(* Logix 5000 AddOnInstructionDefinition export MAS_Yaskawa; software revision 17.00 *)

TYPE Yaskawa_EIP_Servo :   // Yaskawa SigmaLogic Axis Structure v2.4.0
STRUCT
   O : Yaskawa_OUT_to_Servo;
   I : Yaskawa_IN_from_Servo;
   AOI_SB : Yaskawa_AOI_Status_Bits;
END_STRUCT
END_TYPE

TYPE Yaskawa_OUT_to_Servo :   // Structure of data sent out to the Yaskawa SigmaLogic controller v2.4.0
STRUCT
   b00_ServoOn : BOOL;   // Servo On
   b01_Stop : BOOL;   // Stops All Current Motion in Progress
   b02_Home : BOOL;   // Start Homing Process
   b03_MoveStart1 : BOOL;   // Start Current Motion
   b06_SuperImpose : BOOL;
   b07_ServoAlarmReset : BOOL;   // Servo Alarm Reset
   b08_ControllerAlarmReset : BOOL;   // SigmaLogic Alarm Reset
   b09_MoveStart2 : BOOL;   // Start Second Motion (Blended Move)
   b10_MoveAbort : BOOL;   // Abort Current Move
   b11_MovePause : BOOL;   // Pause Current Move
   b12_SeqPause : BOOL;   // Indexing Sequence Pause
   b13_SeqResume : BOOL;   // Indexing Sequence Resume
   b14_SeqCancel : BOOL;   // Indexing Sequence Cancel
   b15_AbsEncoderReset : BOOL;   // Absolute Encoder Reset
   b16_SeqStart : BOOL;   // Start Indexing Sequence
   b17_SeqEditSpeed : BOOL;   // Enter Edit Speed
   b18_SeqEditDistance : BOOL;   // Enter Distance Edit
   b19_PLSEnable : BOOL;   // Enable PLS execution
   b20_PLSActivateOutput1 : BOOL;   // Activate PLS output1 switch logic
   b21_PLSActivateOutput2 : BOOL;   // Activate PLS output2 switch logic
   b22_PLSActivateOutput3 : BOOL;   // Activate PLS output3 switch logic
   b23_PLSActivateOutput4 : BOOL;   // Activate PLS output4 switch logic
   b24_SetClock : BOOL;   // Set the remote controller clock with data provided by the PLC
   RebootController : BOOL;
   UseExternalEncoder : BOOL;   // Use External Encoder when executing MAHSP_Yaskawa
   b32_HeatbeatAnswer : BOOL;   // Heartbeat Answer
   BrakeBypassRequest : BOOL;
   SetFwdTorqueLimit : BOOL;
   SetRevTorqueLimit : BOOL;
   TorqueLimit : DINT;
   TorqueRamp : DINT;
   HomeMethod : INT;
   HomeSpeed : DINT;
   HomeAccDec : DINT;   // Home Move Acceleration/Deceleration Rate
   HomeBackOffDistance : DINT;
   HomeCreepSpeed : DINT;
   HomeCreepDistanceLimit : DINT;
   HomeCreepTimeLimit : DINT;
   HomeOffsetDistance : DINT;
   HomeOffsetSpeed : DINT;
   HomePostion : DINT;
   HomeTorque : DINT;
   HomeInputNo : DINT;
   HomeApproachTimeLimit : DINT;
   HomeApproachDistLimit : DINT;
   HomeDirection : INT;
   HomeSwitchMode : INT;
   MoveType : INT;
   MoveDirection : INT;
   MoveAccel1 : DINT;
   MoveAccel2 : DINT;
   MoveDecel1 : DINT;
   MoveDecel2 : DINT;
   MoveSpeed1 : DINT;
   MoveSpeed2 : DINT;
   MoveDistance1 : DINT;
   MoveDistance2 : DINT;
   MovePosition1 : DINT;
   MovePosition2 : DINT;
   RegistrationDistance : DINT;
   GearNumerator : DINT;
   GearDenominator : DINT;
   SuperImposeDistance : DINT;
   Resolution : INT;
   RegistrationDirection : INT;
   TuningLevel : INT;
   SequenceStep : INT;   // Staring Sequence Step Number
   SequenceEditStep : INT;   // Sequence Step Number to Edit
   FlagCommandBits1 : DINT;   // Flag Commands. 1..64 are General Flags, Bits 0..31 correspond to Flag 1..32
   FlagCommandBits2 : DINT;   // Flag Commands cont. 1..64 are General Flags, Bits 0..31 correspond to Flag 33..64
   DigitalOutCommandBits : DINT;   // Digital Output commands. Bits 0-7 correspond to CN13 Digital Outputs 0-7, used as Flag 73-80. Bits 8-10 correspond to CN1 Digital Outputs 0-2 used as Flag 88-90"
   SequenceEditSpeed : DINT;
   SequenceEditDistance : DINT;
   FeedRateOverride : INT;
   HSI_Enable : BOOL;
   HSI_MoveMode : BOOL;   // 0=Relative; 1=Moves per Cycle
   HSI_CalcMethod : BOOL;   // 0=Accel/Decel; 1=Time
   HSI_MoveDirection : BOOL;   // 0 = Negative; 1 = Positive
   HSI_TriggerFlag : INT;
   HSI_MovingFlag : INT;
   HSI_DwellingFlag : INT;
   HSI_DoneFlag : INT;
   HSI_MoveType : INT;   // 0=Single; 1=Repeat; 2=Repeat "x" times
   HSI_RepeatNumber : INT;
   HSI_Distance : DINT;
   HSI_Speed : DINT;
   HSI_Accel : DINT;
   HSI_MoveTime : DINT;
   HSI_DwellTime : DINT;
   PLS_OutputFlag1 : INT;
   PLS_OutputFlag2 : INT;
   PLS_OutputFlag3 : INT;
   PLS_OutputFlag4 : INT;
   PLS_OnPosition1 : DINT;
   PLS_OffPosition1 : DINT;
   PLS_OnPosition2 : DINT;
   PLS_OffPosition2 : DINT;
   PLS_OnPosition3 : DINT;
   PLS_OffPosition3 : DINT;
   PLS_OnPosition4 : DINT;
   PLS_OffPosition4 : DINT;
   PLS_OnCompensation1 : INT;
   PLS_OffCompensation1 : INT;
   PLS_OnCompensation2 : INT;
   PLS_OffCompensation2 : INT;
   PLS_OnCompensation3 : INT;
   PLS_OffCompensation3 : INT;
   PLS_OnCompensation4 : INT;
   PLS_OffCompensation4 : INT;
   RTC_Year : INT;
   RTC_Month : INT;
   RTC_Day : INT;
   RTC_Hour : INT;
   RTC_Min : INT;
   RTC_Sec : INT;
   StopDecel : DINT;
   AnalogOutput : INT;   // CN13, AO_01 [mV]
END_STRUCT
END_TYPE

TYPE Yaskawa_AOI_Status_Bits :   // Internal bits used to interlock Yaskawa AOI execution. v2.4.0
STRUCT
   MAM : BOOL;   // Move AOI Active
   MAJ : BOOL;   // Jog AOI Active
   MAB : BOOL;   // Blending AOI Active
   MAG : BOOL;   // Gearing AOI Active
   MAHSP : BOOL;   // Home SetPoint AOI Active
   MAH : BOOL;   // Homing AOI Active
   MSQE : BOOL;   // Sequence Edit AOI Active
   MSQR : BOOL;   // Sequence Run AOI Active
   MHSI : BOOL;   // High Speed Index AOI Active
   MSO : BOOL;   // Servo On
   MSF : BOOL;   // Servo Off
   MAFR : BOOL;   // Fault Reset
   MAS : BOOL;   // Servo Abort
   MTRQ : BOOL;   // Torque Mode Active
   MPLS : BOOL;   // PLS Active
   MCLK : BOOL;   // SetClock Active
   MSTL : BOOL;   // Set Torque Limit Active
   AOI_Permissive : BOOL;   // Permissive to Execute an AOI
END_STRUCT
END_TYPE

TYPE Yaskawa_IN_from_Servo :   // Structure of data coming from the Yaskawa SigmaLogic controller. v2.4.0
STRUCT
   AlarmText : STRING;   // ServoPack Alarm Code plus Text Description
   b00_Heartbeat : BOOL;
   b01_Alarm : BOOL;   // ServoPack Alarm
   b02_Warning : BOOL;   // ServoPack Warning
   b03_Ready : BOOL;   // ServoPack Ready
   b04_Enabled : BOOL;   // ServoPack Enabled ("Servo On")
   b05_StopComplete : BOOL;
   b06_HomeComplete : BOOL;
   b07_HomeBusy : BOOL;
   b08_HomeActive : BOOL;
   b09_HomeAborted : BOOL;
   b10_HomeError : BOOL;
   b11_MoveAbsComplete : BOOL;
   b12_MoveAbsBusy : BOOL;
   b13_MoveAbsActive : BOOL;
   b14_MoveAbsAborted : BOOL;
   b15_MoveAbsError : BOOL;
   b16_MoveRelComplete : BOOL;
   b17_MoveRelBusy : BOOL;
   b18_MoveRelActive : BOOL;
   b19_MoveRelAborted : BOOL;
   b20_MoveRelError : BOOL;
   b21_JogAtSpeed : BOOL;
   b22_JogBusy : BOOL;
   b23_JogActive : BOOL;
   b24_JogAborted : BOOL;
   b25_JogError : BOOL;
   b26_GearInSync : BOOL;
   b27_GearBusy : BOOL;
   b28_GearActive : BOOL;
   b29_GearAborted : BOOL;
   b30_GearError : BOOL;
   b32_MoveSuperComplete : BOOL;
   b33_MoveSuperBusy : BOOL;
   b34_MoveSuperActive : BOOL;
   b35_MoveSuperAborted : BOOL;
   b36_MoveSuperError : BOOL;
   b37_PowerCycleRequired : BOOL;
   b38_MoveBlend1Complete : BOOL;
   b39_MoveBlend1Busy : BOOL;
   b40_MoveBlend1Active : BOOL;
   b41_MoveBlend1Abort : BOOL;
   b42_MoveBlend1Error : BOOL;
   b43_MoveBlend2Complete : BOOL;
   b44_MoveBlend2Busy : BOOL;
   b45_MoveBlend2Active : BOOL;
   b46_MoveBlend2Abort : BOOL;
   b47_MoveBlend2Error : BOOL;
   b48_RegComplete : BOOL;
   b49_RegBusy : BOOL;
   b50_RegActive : BOOL;
   b51_RegAborted : BOOL;
   b52_RegError : BOOL;
   b53_ResetAbsEncoderActive : BOOL;
   b54_ResetAbsEncoderBusy : BOOL;
   b55_ResetAbsEncoderDone : BOOL;
   b56_ResetAbsEncoderError : BOOL;
   b57_SeqRunning : BOOL;
   b58_RegSensorNotReached : BOOL;
   b59_SeqEditError : BOOL;
   b60_SeqEditDone : BOOL;
   b61_TorqueAtTorque : BOOL;
   b62_TorqueBusy : BOOL;
   b63_TorqueActive : BOOL;
   b64_TorqueAborted : BOOL;
   b65_TorqueError : BOOL;
   b66_ControllerAlarm : BOOL;
   b67_ApplicationError : BOOL;
   b68_AxisAtStandStill : BOOL;
   b69_TestModeActive : BOOL;
   b70_ServoParamsOK : BOOL;
   b71_SetFwdTorqueLimitDone : BOOL;
   b72_SetRevTorqueLimitDone : BOOL;
   Position : DINT;
   Speed : DINT;
   Torque : DINT;
   HomeErrorID : INT;
   MoveAbsErrorID : INT;
   MoveRelErrorID : INT;
   JogErrorID : INT;
   GearErrorID : INT;
   MoveSuperErrorID : INT;
   ServoAlarmID : INT;
   ServoWarningID : INT;
   ControllerAlarmID : DINT;
   AxisGenAlarmID : DINT;
   MoveBlend1ErrorID : INT;
   MoveBlend2ErrorID : INT;
   ResetAbsEncoderErrorID : INT;
   FunctionBlockErrorID : INT;
   TorqueErrorID : INT;
   RegErrorID : INT;
   SeqCurrentStep : INT;
   FlagStatusBit1 : DINT;   // Flag Status. 1..64 are General Flags, Bits 0..31 correspond to Flag 1..32
   FlagStatusBit2 : DINT;   // Flag Status cont. 1..64 are General Flags, Bits 0..31 correspond to Flag 33..64
   IOStatusBits : DINT;   // Digital IO Status. Bits 0-7, CN13 Inputs 0-7, Used as Flag 65-72. Bits 8-15, CN13 Outputs 0-7, Used as Flag 73-80. Bits 16-22, CN1 Inputs 0-6, Used as Flag 81-87. Bits 23-25, CN1 Outputs 0-4, Used as Flag 88-92.
   HSI_Moving : BOOL;
   HSI_Dwelling : BOOL;
   HSI_Done : BOOL;
   HSI_Busy : BOOL;
   HSI_Error : BOOL;
   HSI_ErrorCode : INT;
   PLS_Running : BOOL;
   PLS_SwitchStatus1 : BOOL;
   PLS_SwitchStatus2 : BOOL;
   PLS_SwitchStatus3 : BOOL;
   PLS_SwitchStatus4 : BOOL;
   PLS_Busy : BOOL;
   PLS_Error : BOOL;
   PLS_ErrorCode : INT;
   SetClock_Done : BOOL;
   SetClock_Busy : BOOL;
   SetClock_Error : BOOL;
   SetClock_ErrorID : INT;
   SoftwareVersion : DINT;
   FirmwareVersion : DINT;
   CommandedPos : DINT;
   CommandedPosNonCyc : DINT;
   CommandedSpeed : DINT;
   Clock_Year : INT;
   Clock_Month : INT;
   Clock_Day : INT;
   Clock_Hour : INT;
   Clock_Minute : INT;
   Clock_Second : INT;
   AnalogInput : REAL;   // CN13, AI_01 [v]
   BrakeBypassActive : BOOL;
   ForwardTorqueLimit : DINT;
   ReverseTorqueLimit : DINT;
END_STRUCT
END_TYPE

ADD_ON_INSTRUCTION MAS_Yaskawa   (* revision 2.4 0, vendor Yaskawa America, Inc., ExecuteEnableInFalse *)
// Motion Axis Stop
// Revision note:
// 2.4.0: No functional change
// 2.3.1: Moved unlatch of AOI_ON_LOCAL to bottom of EnableInFalse routine so that outputs will be on for at least 1 scan if one-shot on EN is used.
// 2.3.0: No functional change
// 2.0.0: Added IP output for stopping in progress. Improved output operation. Improved interlocking with embedded code.
// 1.2.0: No functional change.
// Initial Release 9/10/2014
// Help:
// This AOI stops any motion in progress on the servo axis on the rising edge of the EnableIN input. The Deceleration rate specified with this AOI will be used during stopping. If Deceleration is left at zero, the rate will default to 1000 units/s/s
VAR_IN_OUT
   Axis : Yaskawa_EIP_Servo; {required}
END_VAR
VAR_INPUT
   Deceleration : REAL; {required}   // The Deceleration rate used during stopping.
END_VAR
VAR_OUTPUT
   EN : BOOL; {visible}   // The AOI is Active
   IP : BOOL; {visible}   // The axis is in the process of stopping
   PC : BOOL; {visible}   // Motion is successfully stopped/aborted
END_VAR
VAR
   AOI_ON_LOCAL : BOOL;
   ScaleFactor : REAL;
   Finished : BOOL;   // The Function is finished
END_VAR

ROUTINE EnableInFalse   (* ladder *)
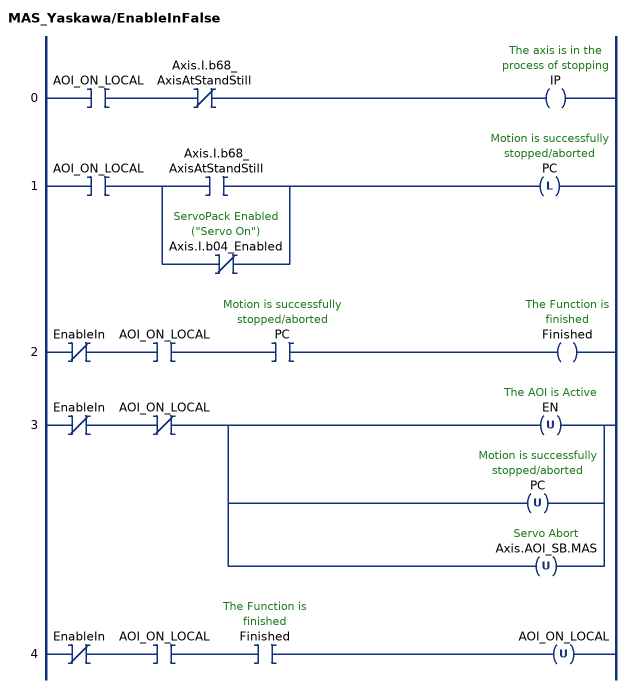
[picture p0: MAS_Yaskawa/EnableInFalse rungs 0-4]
   0: XIC(AOI_ON_LOCAL)XIO(Axis.I.b68_AxisAtStandStill)OTE(IP);
   1: XIC(AOI_ON_LOCAL)[XIC(Axis.I.b68_AxisAtStandStill) ,XIO(Axis.I.b04_Enabled) ]OTL(PC);
   2: XIO(EnableIn)XIC(AOI_ON_LOCAL)XIC(PC)OTE(Finished);
   3: XIO(EnableIn)XIO(AOI_ON_LOCAL)[OTU(EN) ,OTU(PC) ,OTU(Axis.AOI_SB.MAS) ];
   4: XIO(EnableIn)XIC(AOI_ON_LOCAL)XIC(Finished)OTU(AOI_ON_LOCAL);
END_ROUTINE

ROUTINE Logic   (* ladder *)
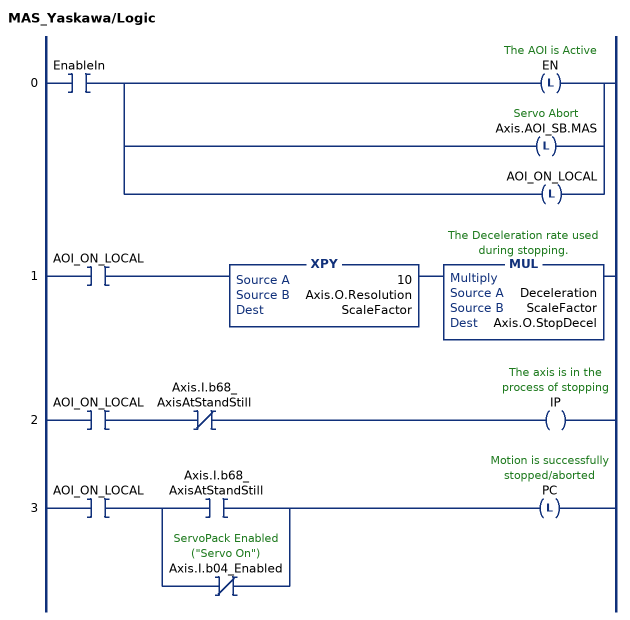
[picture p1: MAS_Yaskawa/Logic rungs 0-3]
   0: XIC(EnableIn)[OTL(EN) ,OTL(Axis.AOI_SB.MAS) ,OTL(AOI_ON_LOCAL) ];
   1: XIC(AOI_ON_LOCAL)XPY(10,Axis.O.Resolution,ScaleFactor)MUL(Deceleration,ScaleFactor,Axis.O.StopDecel);
   2: XIC(AOI_ON_LOCAL)XIO(Axis.I.b68_AxisAtStandStill)OTE(IP);
   3: XIC(AOI_ON_LOCAL)[XIC(Axis.I.b68_AxisAtStandStill) ,XIO(Axis.I.b04_Enabled) ]OTL(PC);
END_ROUTINE
END_ADD_ON_INSTRUCTION
